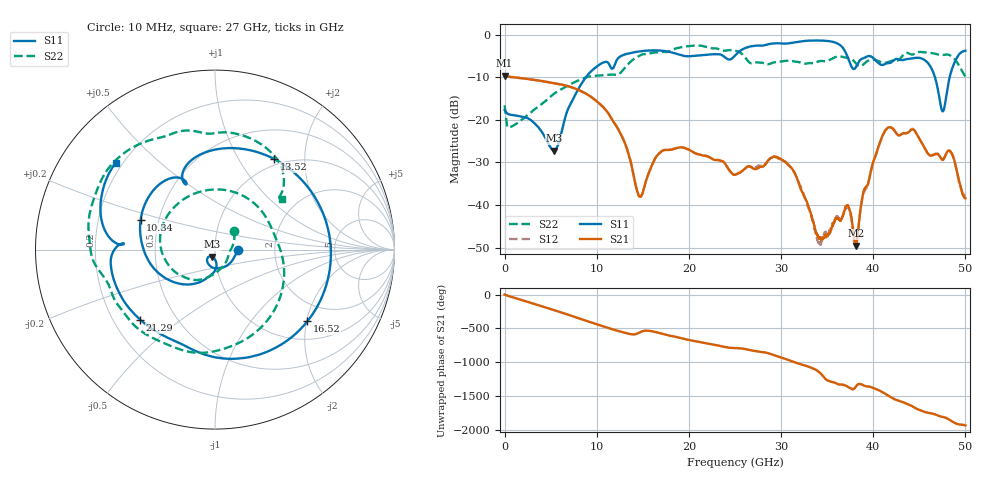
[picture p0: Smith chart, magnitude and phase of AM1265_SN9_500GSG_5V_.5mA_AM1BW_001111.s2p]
!Keysight Technologies,N5245B,MY58422270,A.16.20.02
!Date: Thursday, March 05, 2026 00:46:48
!Correction: S11(C  2-Port  )
!S21(C  2-Port  )
!S12(C  2-Port  )
!S22(C  2-Port  )
!S2P File: Measurements: S11, S21, S12, S22:
# Hz S  dB  R 50
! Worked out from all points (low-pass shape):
!   3201 points, 10 MHz to 50 GHz, reference 50 ohm
!   highest |S21| = -9.69 dB at 10 MHz (marker M1); lowest = -49.6 dB at 38.11 GHz (marker M2)
!   |S21| within 3 dB of the highest: start of sweep to 7.671 GHz
!   lowest |S11| = -27.3 dB at 5.384 GHz (marker M3), VSWR 1.09, Z = 48.2 - j3.85 ohm
!   |S11| at or under -10 dB: start of sweep to 8.844 GHz; 46.7 GHz to 48.29 GHz (1.599 GHz wide, 3.37 % of centre)
!   |S22| runs from -21.8 to -2.5 dB; largest |S21 - S12| = 0.0021
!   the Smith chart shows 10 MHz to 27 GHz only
!   S11 on the Smith chart (normalised r, x): 10 MHz: 1.30, -0.01; 10.34 GHz: 0.39, +0.16; 13.52 GHz: 0.90, +1.43; 16.52 GHz: 1.46, -2.02; 21.29 GHz: 0.31, -0.36; 27 GHz: 0.17, +0.36
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1e7  -17.72 -1.9  -9.69 2.4  -9.67 2.4  -16.63 43.7
2.290794e9  -19.50 -83.0  -10.37 -96.9  -10.37 -96.8  -19.31 -70.6
5.383925e9  -27.30 -112.7  -11.43 131.4  -11.43 131.4  -13.86 -123.2
8.352081e9  -11.53 -133.4  -13.32 -2.5  -13.31 -2.4  -10.45 179.6
1.033606e10  -7.01 158.2  -16.28 -92.4  -16.28 -92.4  -9.60 117.0
1.352292e10  -4.40 56.8  -28.53 139.9  -28.48 139.7  -6.68 -41.8
1.472581e10  -3.93 16.9  -38.11 164.7  -38.03 164.4  -4.88 -92.1
1.652232e10  -3.72 -37.8  -28.50 161.8  -28.47 162.0  -4.19 -141.9
1.667854e10  -3.73 -42.3  -28.11 156.2  -28.09 156.3  -4.20 -145.1
2.128699e10  -4.87 -136.8  -28.26 15.6  -28.24 15.6  -2.62 133.7
2.5005e10  -4.92 175.4  -32.92 -68.2  -32.85 -68.1  -3.77 70.4
2.70046e10  -2.67 138.9  -31.49 -110.1  -31.31 -111.2  -6.66 37.0
3.069136e10  -2.08 78.6  -30.36 118.4  -30.23 118.6  -6.15 -55.7
3.334708e10  -1.41 35.6  -42.83 -5.9  -43.07 -2.2  -6.71 -133.1
3.422191e10  -1.39 20.5  -47.72 -76.2  -49.14 -83.9  -6.22 -152.4
3.667454e10  -3.04 -30.7  -42.71 108.1  -42.70 106.5  -5.24 158.5
3.811175e10  -7.68 -24.0  -49.59 77.2  -49.56 71.1  -6.74 133.3
4.167354e10  -6.70 -53.9  -21.79 -58.4  -21.86 -57.8  -6.42 109.8
4.51416e10  -5.54 -100.9  -24.94 84.9  -24.93 85.1  -4.09 73.5
4.656319e10  -9.14 -149.8  -28.22 33.5  -28.12 32.3  -4.44 54.2
4.771921e10  -17.09 66.7  -28.98 -15.0  -28.86 -14.3  -4.74 41.6
5e10  -3.79 -71.0  -38.46 -136.7  -37.62 -129.0  -9.83 8.9
